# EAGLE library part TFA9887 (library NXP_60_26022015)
Short Description AAL Eindhoven MK
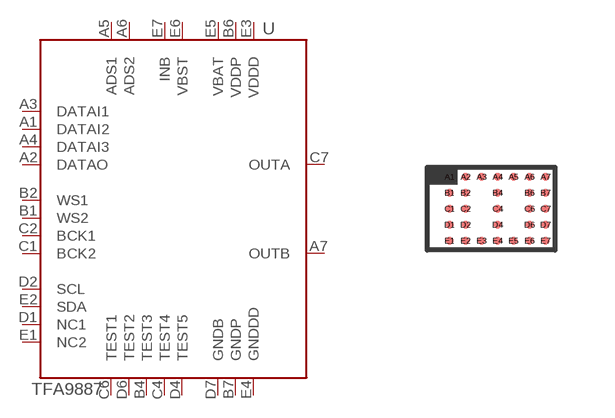
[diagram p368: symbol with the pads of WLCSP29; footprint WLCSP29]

Designator prefix U

## TFA9887  [WLCSP29]
A1  DATAI2  in
A2  DATAO  out
A3  DATAI1  in
A4  DATAI3  in
A5  ADS1  in
A6  ADS2  in
A7  OUTB  out
B1  WS2  in
B2  WS1  in
B4  TEST3  in
B6  VDDP  pwr
B7  GNDP  pwr
C1  BCK2  in
C2  BCK1  in
C4  TEST4  in
C6  TEST1  in
C7  OUTA  out
D1  NC1
D2  SCL
D4  TEST5  in
D6  TEST2  in
D7  GNDB  pwr
E1  NC2
E2  SDA
E3  VDDD  pwr
E4  GNDDD  pwr
E5  VBAT  pwr
E6  VBST  pwr
E7  INB  pwr

## Footprint WLCSP29 (pad centres in mm)
based on Intersil Technical Brief 451
smd 0.2 x 0.2: A1 -1.04,0.797; A2 -0.639,0.797; A3 -0.239,0.797; A4 0.161,0.797; A5 0.56,0.797; A6 0.961,0.797; A7 1.361,0.797; B1 -1.04,0.398; B2 -0.639,0.398; B4 0.161,0.398; B6 0.961,0.398; B7 1.361,0.398; C1 -1.04,-0.003; C2 -0.639,-0.003; C4 0.161,-0.003; C6 0.961,-0.003; C7 1.361,-0.003; D1 -1.04,-0.403; D2 -0.639,-0.403; D4 0.161,-0.403; D6 0.961,-0.403; D7 1.361,-0.403; E1 -1.04,-0.802; E2 -0.639,-0.802; E3 -0.239,-0.802; E4 0.161,-0.802; E5 0.56,-0.802; E6 0.961,-0.802; E7 1.361,-0.802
